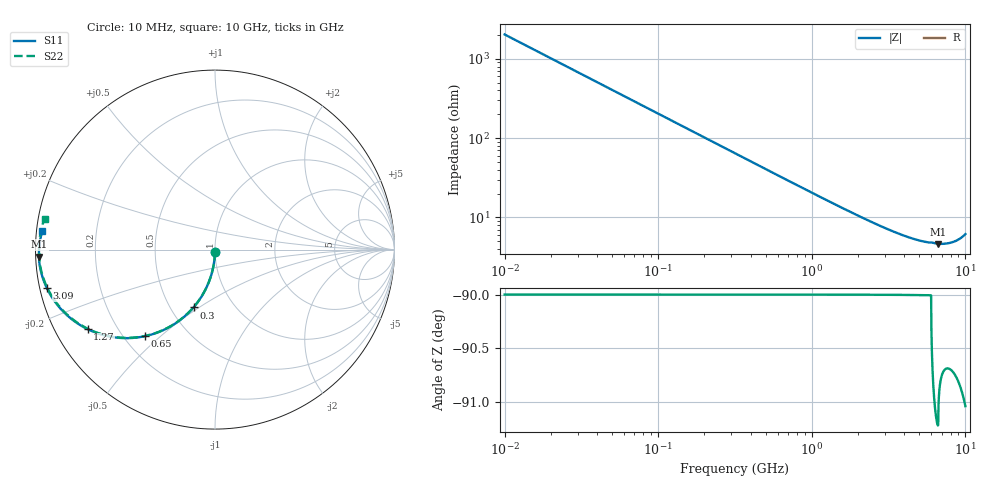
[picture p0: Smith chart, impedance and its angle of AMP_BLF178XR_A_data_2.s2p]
! Created Wed Jun 13 16:07:46 2012
# ghz S ma R 50
! 2 Port Network Data from SP1.SP block
! freq  magS11  angS11  magS21  angS21  magS12  angS12  magS22  angS22
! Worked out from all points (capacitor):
!   1000 points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, 10 MHz to 10 GHz, reference 50 ohm
!   read as one part in shunt: C = 7.83 pF near 60 MHz
!   lowest |Z| = 4.62 ohm at 6.66 GHz (marker M1)
!   S11 on the Smith chart (normalised r, x): 10 MHz: 1.00, -0.02; 300 MHz: 0.65, -0.47; 650 MHz: 0.28, -0.45; 1.27 GHz: 0.10, -0.28; 3.09 GHz: 0.02, -0.11; 10 GHz: 0.02, +0.05
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0.01  0.01221 -90.7  0.9999 -0.7  0.9999 -0.7  0.01221 -90.7
0.04  0.04879 -92.8  0.9988 -2.8  0.9988 -2.8  0.04879 -92.8
0.07  0.08517 -94.9  0.9964 -5.0  0.9964 -5.0  0.08517 -95.0
0.09  0.1092 -96.4  0.994 -6.4  0.994 -6.4  0.1092 -96.4
0.11  0.1331 -97.8  0.9911 -7.8  0.9911 -7.8  0.1331 -97.8
0.15  0.1801 -100.5  0.9836 -10.5  0.9836 -10.5  0.1801 -100.6
0.19  0.2259 -103.2  0.9741 -13.3  0.9741 -13.3  0.2259 -103.3
0.24  0.2811 -106.5  0.9597 -16.6  0.9597 -16.6  0.2811 -106.6
0.3  0.3437 -110.4  0.9391 -20.4  0.9391 -20.4  0.3437 -110.5
0.45  0.4809 -119.2  0.8768 -29.2  0.8768 -29.2  0.4809 -119.3
0.65  0.6203 -128.9  0.7844 -39.0  0.7844 -39.0  0.6203 -129.1
0.95  0.7549 -139.9  0.6559 -50.0  0.6559 -50.0  0.7549 -140.1
1.27  0.8369 -148.0  0.5473 -58.2  0.5473 -58.2  0.8369 -148.3
1.68  0.8946 -155.1  0.4469 -65.3  0.4469 -65.3  0.8946 -155.5
2.27  0.9356 -161.5  0.3531 -71.8  0.3531 -71.8  0.9356 -162.1
3.09  0.9608 -167.0  0.2771 -77.5  0.2771 -77.5  0.9608 -167.9
3.34  0.9652 -168.3  0.2613 -78.7  0.2613 -78.7  0.9652 -169.2
5.01  0.9794 -174.0  0.2017 -84.7  0.2017 -84.7  0.9794 -175.4
6.66  0.9801 -177.7  0.1826 -89.9  0.1826 -89.9  0.9785 -179.8
6.67  0.9803 -177.8  0.1827 -89.9  0.1827 -89.9  0.9789 -179.8
8.34  0.979 178.6  0.1936 -93.6  0.1936 -93.6  0.9781 175.7
10  0.967 173.9  0.2401 -99.3  0.2401 -99.3  0.9655 169.7
